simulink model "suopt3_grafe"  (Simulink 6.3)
settings: Solver=ode4  StartTime=0.0  StopTime=5.0  FixedStep=0.01  RelTol=1e-7
undefined symbols (not defined in the file or in its folder): sgn

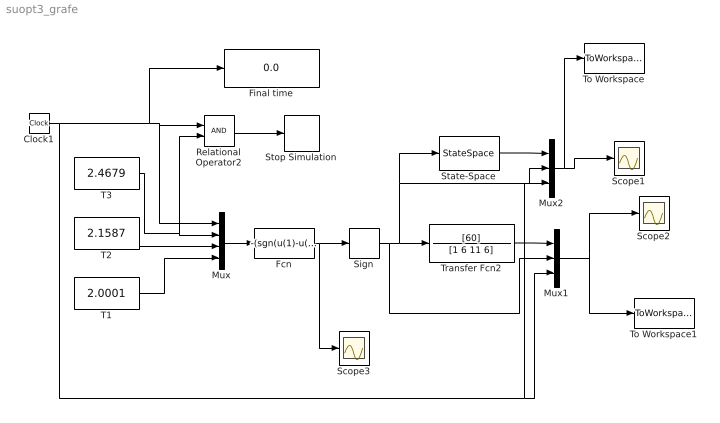
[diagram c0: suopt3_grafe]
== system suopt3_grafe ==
  Clock1 : Clock
  Fcn : Fcn  Expr=-(sgn(u(1)-u(2))*sgn(u(1)-u(3))*sgn(u(1)-u(4)))
  Final time : Display
  Mux : Mux
  Mux1 : Mux  Inputs=3
  Mux2 : Mux  Inputs=3
  Relational Operator2 : RelationalOperator
  Scope1 : Scope
  Scope2 : Scope
  Scope3 : Scope
  Sign : Signum
  State-Space : StateSpace  A=[0 1 0;0 0 1;-6 -11 -6]  B=[0;0;60]  C=[1 0 0;0 1 0;0 0 1]  D=[0;0;0]
  Stop Simulation : Stop
  T1 : Constant  Value=2.0001
  T2 : Constant  Value=2.1587
  T3 : Constant  Value=2.4679
  To Workspace : ToWorkspace  VariableName=simout  SampleTime=-1  SaveFormat=Array
  To Workspace1 : ToWorkspace  VariableName=simout1  SampleTime=-1  SaveFormat=Array
  Transfer Fcn2 : TransferFcn  Numerator=[60]  Denominator=[1 6 11 6]
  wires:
  T3/1 -> Mux/2, Relational Operator2/2
  T2/1 -> Mux/3
  T1/1 -> Mux/4
  Mux/1 -> Fcn/1
  Fcn/1 -> Sign/1, Scope3/1
  Sign/1 -> Mux1/2, Transfer Fcn2/1, State-Space/1, Mux2/2
  Clock1/1 -> Mux/1, Relational Operator2/1, Final time/1, Mux1/3, Mux2/3
  Relational Operator2/1 -> Stop Simulation/1
  Transfer Fcn2/1 -> Mux1/1
  Mux1/1 -> Scope2/1, To Workspace1/1
  State-Space/1 -> Mux2/1
  Mux2/1 -> Scope1/1, To Workspace/1
